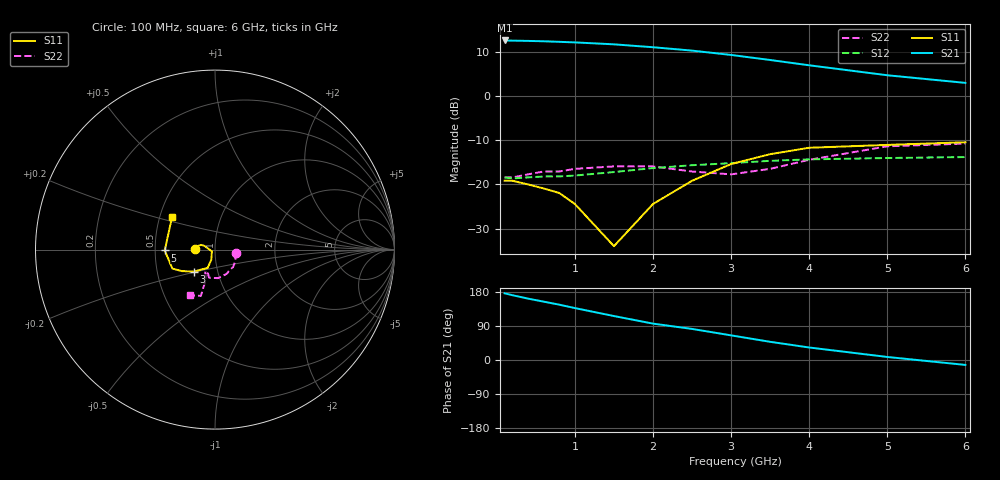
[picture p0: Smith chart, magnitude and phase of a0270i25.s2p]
!  MSA-0270 S AND NOISE PARAMETERS
!  Id=25mA  LAST UPDATED 07-22-92
# ghz s ma r 50
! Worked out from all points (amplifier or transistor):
!   14 points, 100 MHz to 6 GHz, reference 50 ohm
!   highest |S21| = 12.6 dB at 100 MHz (marker M1)
!   |S21| within 3 dB of that: start of sweep to 2.857 GHz
!   unconditionally stable (mu >= 1): start of sweep to end of sweep
!   at 400 MHz: K = 1.20, MAG = 12.7 dB, |S12| = -18.4 dB
!   at 2 GHz: K = 1.15, MAG = 11.3 dB, |S12| = -16.3 dB
!   at 6 GHz: K = 1.54, MAG = 4.1 dB, |S12| = -13.8 dB
!   lowest NFmin = 6.00 dB at 100 MHz
!   S11 on the Smith chart (normalised r, x): 100 MHz: 0.80, +0.00; 3 GHz: 0.77, -0.19; 5 GHz: 0.56, -0.01; 6 GHz: 0.58, +0.23
0.1  0.11 179.0  4.26 176.0  0.12 1.0  0.12 -8.0
0.2  0.11 174.0  4.24 171.0  0.117 3.0  0.12 -15.0
0.4  0.1 169.0  4.21 162.0  0.12 4.0  0.13 -30.0
0.6  0.09 165.0  4.17 154.0  0.123 5.0  0.14 -44.0
0.8  0.08 161.0  4.11 146.0  0.123 7.0  0.14 -55.0
1  0.06 161.0  4.05 137.0  0.126 9.0  0.15 -64.0
1.5  0.02 -150.0  3.85 116.0  0.138 11.0  0.16 -84.0
2  0.06 -110.0  3.57 96.0  0.153 11.0  0.16 -102.0
2.5  0.11 -112.0  3.27 82.0  0.165 14.0  0.14 -106.0
3  0.17 -134.0  2.92 65.0  0.174 12.0  0.13 -114.0
3.5  0.22 -147.0  2.56 48.0  0.185 6.0  0.15 -111.0
4  0.26 -156.0  2.23 33.0  0.192 3.0  0.19 -107.0
5  0.28 -179.0  1.72 8.0  0.199 -6.0  0.27 -107.0
6  0.3 143.0  1.41 -13.0  0.204 -14.0  0.29 -119.0
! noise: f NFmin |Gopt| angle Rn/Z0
0.1  6  0.08  2  1.14
0.5  6.3  0.08  11  1.14
1  6.5  0.07  19  1.13
2  6.9  0.06  44  1.09
